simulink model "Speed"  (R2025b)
settings: Solver=FixedStepAuto  StartTime=0.0  StopTime=10.0  FixedStep=1e-4  RelTol=1e-3
undefined symbols (not defined in the file): case, constant, DiscIntNeverNeededParam, flux, lambda_pm, linkage, Permanent, Pn, sigbuilder_block, spd_ki, spd_kp
libraries: slpidlib x3, mcbplantlib x1, autolibpmsmexterior x1

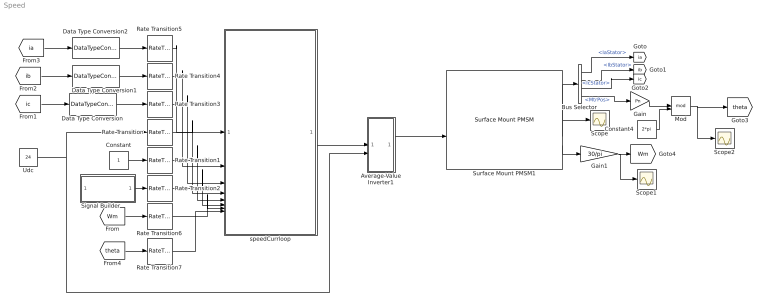
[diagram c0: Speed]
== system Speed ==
  Average-Value Inverter1 : Subsystem
  Bus Selector : BusSelector  OutputSignals=IaStator,IbStator,IcStator,MtrPos
  Constant : Constant
  Constant4 : Constant  Value=2*pi  OutDataTypeStr=Inherit: Inherit via back propagation
  Data Type Conversion : DataTypeConversion  OutDataTypeStr=single
  Data Type Conversion1 : DataTypeConversion  OutDataTypeStr=single
  Data Type Conversion2 : DataTypeConversion  OutDataTypeStr=single
  Gain : Gain  Gain=Pn
  Gain1 : Gain  Gain=30/pi  OutDataTypeStr=single
  Mod : Math  Operator=mod
  Rate Transition{,1..7} (8 alike) : RateTransition
  Scope : Scope
  Scope1 : Scope
  Scope2 : Scope
  Signal Builder : Subsystem  Tag=STV Subsys  LoadFcn=sigbuilder_block('load');  StartFcn=sigbuilder_block('start');  StopFcn=sigbuilder_block('stop');  ClipboardFcn=sigbuilder_block('clipboard');  mask(Sigbuilder block){tuvar=[0:10]}
      mask init:
      | if ~strcmp(get_param(bdroot(gcb),'SimulationStatus'),'stopped'),tuvar = sigbuilder_block('maskInit'); end
  Surface Mount PMSM1 : autolibpmsmexterior/Surface Mount PMSM  port_config=Torque  sim_type=Continuous  Ts=0.001  P=Pn  Rs=Rs  Ldq_=L  KConstText=Permanent flux linkage constant (lambda_pm):  lambda_pm=flux  Ke=159.9771  Kt=1.323  mechanical=[75e-6,8e-5,0]  idq0=[0 0]  theta_init=0  omega_init=0  KConst=0.2205  lambda_pm_calc=0.2205  RefBlkName='autolibpmsmexterior/Surface Mount PMSM'  aMode=5  Ldq="[0.0017      0.0017]"
  Udc : Constant  Value=24
  speedCurrloop : Subsystem
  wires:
  [ia] -> Data Type Conversion2/1
  [ib] -> Data Type Conversion1/1
  [ic] -> Data Type Conversion/1
  Data Type Conversion2/1 -> Rate Transition5/1
  Data Type Conversion1/1 -> Rate Transition4/1
  Data Type Conversion/1 -> Rate Transition3/1
  Udc/1 -> Average-Value Inverter1/2(udc), Rate Transition/1
  Average-Value Inverter1/1(vabc) -> Surface Mount PMSM1/2
  Surface Mount PMSM1/2 -> Scope/1
  Surface Mount PMSM1/1 -> Bus Selector/1
  Bus Selector/1 -> [ia]  "<IaStator>"
  Bus Selector/2 -> [ib]  "<IbStator>"
  Bus Selector/3 -> [ic]  "<IcStator>"
  Bus Selector/4 -> Gain/1  "<MtrPos>"
  Gain/1 -> Mod/1
  Constant4/1 -> Mod/2
  Mod/1 -> Scope2/1, [theta]
  Rate Transition5/1 -> speedCurrloop/1(ia)
  Rate Transition4/1 -> speedCurrloop/2(ib)
  Rate Transition3/1 -> speedCurrloop/3(ic)
  Rate Transition/1 -> speedCurrloop/4(v_bus)
  Constant/1 -> Rate Transition1/1
  speedCurrloop/1(IABC1) -> Average-Value Inverter1/1(Dutyln)
  Rate Transition1/1 -> speedCurrloop/5(Motor_OnOff)
  Rate Transition2/1 -> speedCurrloop/6(SpeedRef)
  Rate Transition6/1 -> speedCurrloop/7(SpeedFd)
  Signal Builder/1(Signal 1) -> Rate Transition2/1
  Surface Mount PMSM1/3 -> Gain1/1
  Gain1/1 -> Scope1/1, [Wm]
  [Wm] -> Rate Transition6/1
  Rate Transition7/1 -> speedCurrloop/8(theta)
  [theta] -> Rate Transition7/1

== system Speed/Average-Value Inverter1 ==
  Dutyln : Inport
  udc : Inport  Port=2
  Average-Value Inverter : mcbplantlib/Average-Value Inverter
  Duty : Subsystem
  vabc : Outport
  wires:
  Dutyln/1 -> Duty/1(Dutyln)
  Duty/1(DutyOut) -> Average-Value Inverter/1
  udc/1 -> Average-Value Inverter/2
  Average-Value Inverter/1 -> vabc/1

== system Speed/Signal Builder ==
  Demux : Demux  Tag=STV Demux  Outputs=1
  FromWs : FromWorkspace  Tag=STV FromWs  VariableName=tuvar
  Signal 1 : Outport  Tag=STV Outport
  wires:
  FromWs/1 -> Demux/1
  Demux/1 -> Signal 1/1

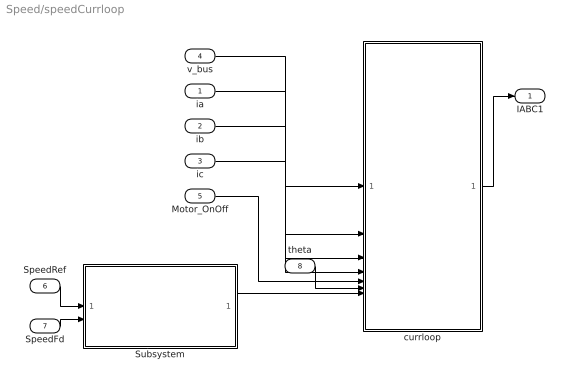
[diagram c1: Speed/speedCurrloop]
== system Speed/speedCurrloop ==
  ia : Inport
  ib : Inport  Port=2
  ic : Inport  Port=3
  v_bus : Inport  Port=4
  Motor_OnOff : Inport  Port=5
  SpeedRef : Inport  Port=6
  SpeedFd : Inport  Port=7
  theta : Inport  Port=8
  Subsystem : Subsystem
  currloop : Subsystem
  IABC1 : Outport
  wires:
  ic/1 -> currloop/4(ic)
  Subsystem/1(iq_ref) -> currloop/7(iq_ref)
  v_bus/1 -> currloop/1(v_bus)
  SpeedRef/1 -> Subsystem/1(SpeedRef)
  ib/1 -> currloop/3(ib)
  currloop/1(IABC1) -> IABC1/1
  Motor_OnOff/1 -> currloop/5(Motor_OnOff)
  ia/1 -> currloop/2(ia)
  SpeedFd/1 -> Subsystem/2(SpeedFd)
  theta/1 -> currloop/6(theta)

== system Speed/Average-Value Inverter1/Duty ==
  Dutyln : Inport
  Subsystem : Subsystem
  DutyOut : Outport
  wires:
  Dutyln/1 -> Subsystem/1(Dutyln)
  Subsystem/1(DutyOut) -> DutyOut/1

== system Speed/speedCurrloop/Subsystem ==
  SpeedRef : Inport
  SpeedFd : Inport  Port=2
  PID Controller : slpidlib/PID Controller  Controller=PI  Form=Parallel  TimeDomain=Discrete-time  UseExternalTs=off  SampleTime=-1  IntegratorMethod=Forward Euler  FilterMethod=Forward Euler  ControllerParametersSource=internal  P=spd_kp  I=spd_ki  UseKiTs=off  D=0  UseExternalDerivativeSource=off  N=100  UseFilter=on  TunerSelectOption=Transfer Function Based (PID Tuner App)  InitialConditionSource=internal  InitialConditionForIntegrator=0  InitialConditionForFilter=0  DifferentiatorICPrevScaledInput=0  ExternalReset=none  TrackingMode=off  Kt=1  LimitOutput=on  SatLimitsSource=internal  UpperSaturationLimit=3  LowerSaturationLimit=-3  LinearizeAsGain=on  AntiWindupMode=clamping  Kb=1  LimitIntegrator=off  UpperIntegratorSaturationLimit=inf  LowerIntegratorSaturationLimit=-inf  POutMin=[]  POutMax=[]  IOutMin=[]  IOutMax=[]  DOutMin=[]  DOutMax=[]  NOutMin=[]  NOutMax=[]  SumOutMin=[]  SumOutMax=[]  SaturationOutMin=[]  SaturationOutMax=[]  PParamMin=[]  PParamMax=[]  IParamMin=[]  IParamMax=[]  DParamMin=[]  DParamMax=[]  NParamMin=[]  NParamMax=[]  KbParamMin=[]  KbParamMax=[]  KtParamMin=[]  KtParamMax=[]  KbOutMin=[]  KbOutMax=[]  KtOutMin=[]  KtOutMax=[]  IntegratorOutMin=[]  IntegratorOutMax=[]  FilterOutMin=[]  FilterOutMax=[]  SumI1OutMin=[]  SumI1OutMax=[]  SumI2OutMin=[]  SumI2OutMax=[]  SumI3OutMin=[]  SumI3OutMax=[]  SumI4OutMin=[]  SumI4OutMax=[]  SumDOutMin=[]  SumDOutMax=[]  DifferentiatorOutMin=[]  DifferentiatorOutMax=[]  FilterDiffOutCoefMin=[]  FilterDiffOutCoefMax=[]  ReciprocalOutMin=[]  ReciprocalOutMax=[]  SumDenOutMin=[]  SumDenOutMax=[]  SumNumOutMin=[]  SumNumOutMax=[]  DivideOutMin=[]  DivideOutMax=[]  UdiffTsProdOutMin=[]  UdiffTsProdOutMax=[]  NTsProdOutMin=[]  NTsProdOutMax=[]  UintegralTsProdOutMin=[]  UintegralTsProdOutMax=[]  UngainTsProdOutMin=[]  UngainTsProdOutMax=[]  ClampingZeroOutDataTypeStr=Inherit: Inherit via back propagation  ClampingZeroOutMin=[]  ClampingZeroOutMax=[]  FilterDenConstantOutDataTypeStr=Inherit: Inherit via back propagation  FilterDenConstantOutMin=[]  FilterDenConstantOutMax=[]  PCopyOutDataTypeStr=Inherit: Inherit via back propagation  PCopyOutMin=[]  PCopyOutMax=[]  NCopyOutDataTypeStr=Inherit: Inherit via back propagation  NCopyOutMin=[]  NCopyOutMax=[]  IntegratorContinuousStateAttributes=''  IntegratorStateMustResolveToSignalObject=off  IntegratorRTWStateStorageClass=Auto  FilterContinuousStateAttributes=''  FilterStateMustResolveToSignalObject=off  FilterRTWStateStorageClass=Auto  ParallelPVariant=InternalParameters  IdealPVariant=Disabled  IVariant=InternalParameters  DVariant=Disabled  IntegratorVariant=Discrete  SatVariant=Enabled  AWVariant=DiscClampingParallel  PCopyVariant=Disabled  TRVariant=Disabled  FdbkBlocksVariant=Forward  IdealPFdbkVariant=Disabled  SatFdbkVariant=Disabled  DerivativeFilterVariant=Disabled  NVariant=Disabled  NCopyVariant=Disabled_SignalSpec  FilterICVariant=Disabled  IntegratorICVariant=InternalICs  ExternalResetVariant=Disabled  TRSumVariant=Passthrough  SumFdbkVariant=Disabled  SumVariant=Sum_PI  TsampFilterVariant=InternalTs  TsampNgainVariant=Passthrough  TsampIntegralVariant=Disabled_SignalSpec  ExternalSaturationOutDataTypeStr=Inherit: Same as second input  DerivativeSourceVariant=Disabled  PreIntVariant=InternalPreInt
  Sum : Sum  Inputs=|+-
  iq_ref : Outport
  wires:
  Sum/1 -> PID Controller/1
  SpeedRef/1 -> Sum/1
  SpeedFd/1 -> Sum/2
  PID Controller/1 -> iq_ref/1

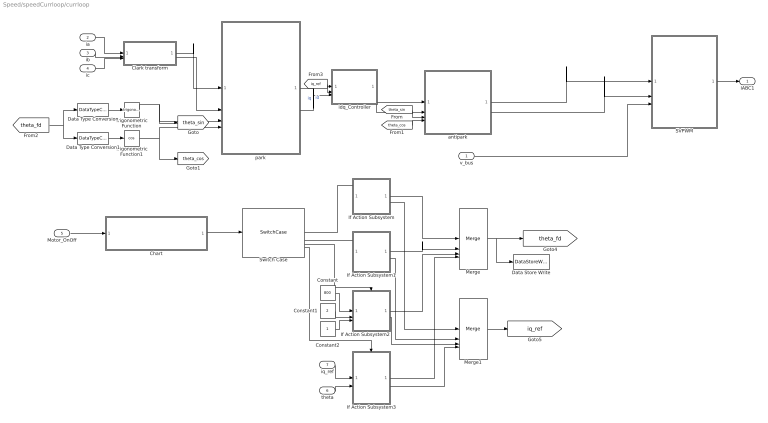
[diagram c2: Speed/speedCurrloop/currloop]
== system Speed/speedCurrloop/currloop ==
  v_bus : Inport
  ia : Inport  Port=2
  ib : Inport  Port=3
  ic : Inport  Port=4
  Motor_OnOff : Inport  Port=5
  theta : Inport  Port=6
  iq_ref : Inport  Port=7
  Chart : Stateflow chart  TreatAsAtomicUnit=on
  Clark transform : Subsystem
  Constant : Constant  Value=800
  Constant1 : Constant  Value=2
  Constant2 : Constant
  Data Store Write : DataStoreWrite  DataStoreName=ThetaOpen  IndexOptions=Index vector (dialog)  Indices=1  OutputSizes=1
  Data Type Conversion : DataTypeConversion  OutDataTypeStr=single
  Data Type Conversion1 : DataTypeConversion  OutDataTypeStr=single
  If Action Subsystem : Subsystem  TreatAsAtomicUnit=on
  If Action Subsystem1 : Subsystem  TreatAsAtomicUnit=on
  If Action Subsystem2 : Subsystem  TreatAsAtomicUnit=on
  If Action Subsystem3 : Subsystem  TreatAsAtomicUnit=on
  Merge : Merge  Inputs=4
  Merge1 : Merge  Inputs=4
  SVPWM : Subsystem
  Switch Case : SwitchCase  CaseConditions={1,2,3,4}  ShowDefaultCase=off
  Trigonometric Function : Trigonometry
  Trigonometric Function1 : Trigonometry  Operator=cos
  antipark : Subsystem
  idq_Controller : Subsystem
  park : Subsystem
  IABC1 : Outport
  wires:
  Clark transform/2(ibeta) -> park/2(ibeta)
  Trigonometric Function1/1 -> [theta_cos], park/4(theta_cos)
  park/1(id) -> idq_Controller/1(id_fdbk)  "id"
  Trigonometric Function/1 -> [theta_sin], park/3(theta_sin)
  idq_Controller/2(uq_ref) -> antipark/2(uq)
  [theta_cos] -> antipark/4(theta_cos)
  Clark transform/1(ialpha) -> park/1(ialpha)
  [theta_fd] -> Data Type Conversion1/1, Data Type Conversion/1
  Data Type Conversion/1 -> Trigonometric Function/1
  park/2(iq) -> idq_Controller/3(iq_fdbk)  "iq"
  [theta_sin] -> antipark/3(theta_sin)
  SVPWM/1(IABC) -> IABC1/1
  antipark/2(ubeta) -> SVPWM/2(Vbeta)
  ic/1 -> Clark transform/3(ic)
  antipark/1(ualpha) -> SVPWM/1(Valpha)
  Data Type Conversion1/1 -> Trigonometric Function1/1
  idq_Controller/1(ud_ref) -> antipark/1(ud)
  v_bus/1 -> SVPWM/3(v_bus)
  ib/1 -> Clark transform/2(ib)
  [iq_ref] -> idq_Controller/2(iq_ref)
  ia/1 -> Clark transform/1(ia)
  If Action Subsystem2/1(theta_fd) -> Merge/3
  Merge/1 -> Data Store Write/1, [theta_fd]
  If Action Subsystem/2(iq_ref) -> Merge1/1
  If Action Subsystem1/1(theta__fd) -> Merge/2
  Switch Case/4 -> If Action Subsystem3/Action
  Constant2/1 -> If Action Subsystem2/3(iq_ref)
  Switch Case/1 -> If Action Subsystem/Action
  If Action Subsystem3/1(theta_fd) -> Merge/4
  If Action Subsystem2/2(iq_fd) -> Merge1/3
  Chart/1(Motor_state) -> Switch Case/1
  Switch Case/3 -> If Action Subsystem2/Action
  Constant/1 -> If Action Subsystem2/1(OPSpd)
  If Action Subsystem1/2(iq_ref) -> Merge1/2
  Merge1/1 -> [iq_ref]
  If Action Subsystem/1(theta_fd) -> Merge/1
  If Action Subsystem3/2(iq_fd) -> Merge1/4
  Switch Case/2 -> If Action Subsystem1/Action
  Constant1/1 -> If Action Subsystem2/2(OPTime)
  Motor_OnOff/1 -> Chart/1(Motor_OnOff)
  iq_ref/1 -> If Action Subsystem3/1(iq_ref)
  theta/1 -> If Action Subsystem3/2(theta)

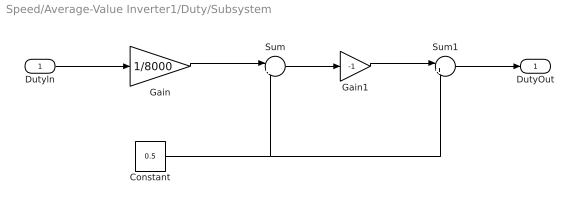
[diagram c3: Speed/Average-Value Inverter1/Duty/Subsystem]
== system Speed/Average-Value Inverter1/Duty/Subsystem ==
  Dutyln : Inport
  Constant : Constant  Value=0.5
  Gain : Gain  Gain=1/8000
  Gain1 : Gain  Gain=-1
  Sum : Sum  Inputs=|+-
  Sum1 : Sum  Inputs=|++
  DutyOut : Outport
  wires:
  Dutyln/1 -> Gain/1
  Constant/1 -> Sum/2, Sum1/2
  Sum1/1 -> DutyOut/1
  Gain/1 -> Sum/1
  Gain1/1 -> Sum1/1
  Sum/1 -> Gain1/1

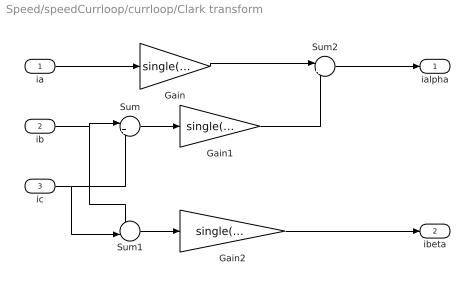
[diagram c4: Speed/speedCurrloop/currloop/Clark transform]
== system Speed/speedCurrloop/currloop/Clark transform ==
  ia : Inport
  ib : Inport  Port=2
  ic : Inport  Port=3
  Gain : Gain  Gain=single(2/3)
  Gain1 : Gain  Gain=single(1/3)
  Gain2 : Gain  Gain=single(sqrt(3)/3)
  Sum : Sum  Inputs=|++
  Sum1 : Sum  Inputs=+-|
  Sum2 : Sum  Inputs=|+-
  ialpha : Outport
  ibeta : Outport  Port=2
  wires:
  ia/1 -> Gain/1
  ib/1 -> Sum1/1, Sum/1
  ic/1 -> Sum1/2, Sum/2
  Sum/1 -> Gain1/1
  Sum1/1 -> Gain2/1
  Gain/1 -> Sum2/1
  Gain1/1 -> Sum2/2
  Gain2/1 -> ibeta/1
  Sum2/1 -> ialpha/1

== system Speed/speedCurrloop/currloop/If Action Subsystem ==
  Action Port : ActionPort  ActionPortLabel=case [ 1 ]:
  Constant : Constant  Value=0
  Constant1 : Constant  Value=0
  theta_fd : Outport
  iq_ref : Outport  Port=2
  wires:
  Constant/1 -> theta_fd/1
  Constant1/1 -> iq_ref/1

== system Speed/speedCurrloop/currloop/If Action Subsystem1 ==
  Action Port : ActionPort  ActionPortLabel=case [ 2 ]:
  Constant : Constant  Value=0
  Constant1 : Constant
  theta__fd : Outport
  iq_ref : Outport  Port=2
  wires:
  Constant/1 -> theta__fd/1
  Constant1/1 -> iq_ref/1

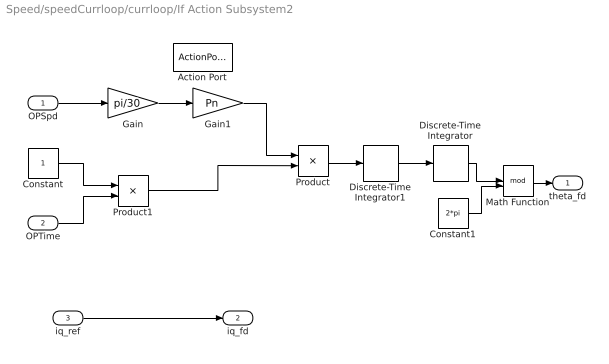
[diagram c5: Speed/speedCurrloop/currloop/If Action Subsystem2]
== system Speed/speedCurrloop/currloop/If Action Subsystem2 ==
  OPSpd : Inport
  OPTime : Inport  Port=2
  iq_ref : Inport  Port=3
  Action Port : ActionPort  ActionPortLabel=case [ 3 ]:
  Constant : Constant
  Constant1 : Constant  Value=2*pi
  Discrete-Time Integrator : DiscreteIntegrator  SampleTime=-1  ICPrevOutput=DiscIntNeverNeededParam  ICPrevScaledInput=DiscIntNeverNeededParam
  Discrete-Time Integrator1 : DiscreteIntegrator  SampleTime=-1  ICPrevOutput=DiscIntNeverNeededParam  ICPrevScaledInput=DiscIntNeverNeededParam
  Gain : Gain  Gain=pi/30  OutDataTypeStr=single
  Gain1 : Gain  Gain=Pn
  Math Function : Math  Operator=mod
  Product : Product
  Product1 : Product  Inputs=*/
  theta_fd : Outport
  iq_fd : Outport  Port=2
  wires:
  OPTime/1 -> Product1/2
  Constant/1 -> Product1/1
  Product/1 -> Discrete-Time Integrator1/1
  Gain/1 -> Gain1/1
  Gain1/1 -> Product/1
  Constant1/1 -> Math Function/2
  OPSpd/1 -> Gain/1
  Discrete-Time Integrator/1 -> Math Function/1
  Discrete-Time Integrator1/1 -> Discrete-Time Integrator/1
  Math Function/1 -> theta_fd/1
  Product1/1 -> Product/2
  iq_ref/1 -> iq_fd/1

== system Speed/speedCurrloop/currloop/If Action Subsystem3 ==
  iq_ref : Inport  SampleTime=1e-4
  theta : Inport  Port=2  SampleTime=1e-4
  Action Port : ActionPort  ActionPortLabel=case [ 4 ]:
  theta_fd : Outport  SampleTime=1e-4
  iq_fd : Outport  Port=2  SampleTime=1e-4
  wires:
  theta/1 -> theta_fd/1
  iq_ref/1 -> iq_fd/1

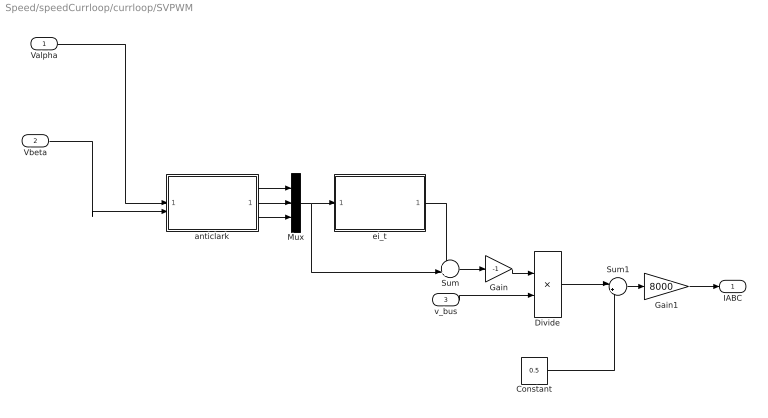
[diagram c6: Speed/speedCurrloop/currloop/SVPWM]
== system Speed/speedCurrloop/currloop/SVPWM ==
  Valpha : Inport
  Vbeta : Inport  Port=2
  v_bus : Inport  Port=3  OutMin=10
  Constant : Constant  Value=0.5
  Divide : Product  Inputs=*/
  Gain : Gain  Gain=-1
  Gain1 : Gain  Gain=8000
  Mux : Mux  Inputs=3
  Sum : Sum  Inputs=++|
  Sum1 : Sum  Inputs=|++
  anticlark : Subsystem
  ei_t : Subsystem
  IABC : Outport
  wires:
  ei_t/1(ei_t1) -> Sum/1
  Gain1/1 -> IABC/1
  anticlark/2(Vb) -> Mux/2
  Vbeta/1 -> anticlark/2(Vbeta)
  Constant/1 -> Sum1/2
  anticlark/3(Vc) -> Mux/3
  Divide/1 -> Sum1/1
  Sum/1 -> Gain/1
  Gain/1 -> Divide/1
  Sum1/1 -> Gain1/1
  anticlark/1(Va) -> Mux/1
  v_bus/1 -> Divide/2
  Mux/1 -> Sum/2, ei_t/1(Vabc)
  Valpha/1 -> anticlark/1(Valpha)

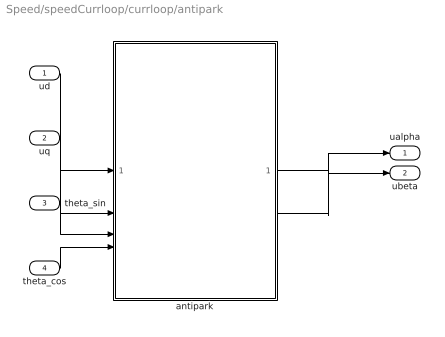
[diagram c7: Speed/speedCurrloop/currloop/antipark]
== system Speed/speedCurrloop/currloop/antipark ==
  ud : Inport
  uq : Inport  Port=2
  theta_sin : Inport  Port=3
  theta_cos : Inport  Port=4
  antipark : Subsystem
  ualpha : Outport
  ubeta : Outport  Port=2
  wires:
  theta_cos/1 -> antipark/4(theta_cos)
  theta_sin/1 -> antipark/3(theta_sin)
  antipark/2(ubeta) -> ubeta/1
  antipark/1(ualpha) -> ualpha/1
  ud/1 -> antipark/1(ud)
  uq/1 -> antipark/2(uq)

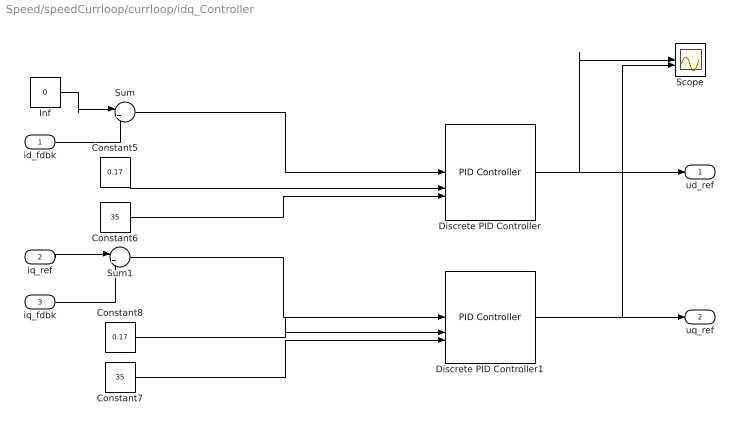
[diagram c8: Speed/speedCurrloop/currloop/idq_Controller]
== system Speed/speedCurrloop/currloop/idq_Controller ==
  id_fdbk : Inport
  iq_ref : Inport  Port=2
  iq_fdbk : Inport  Port=3
  Constant5 : Constant  Value=0.17  OutDataTypeStr=single
  Constant6 : Constant  Value=35  OutDataTypeStr=single
  Constant7 : Constant  Value=35  OutDataTypeStr=single
  Constant8 : Constant  Value=0.17  OutDataTypeStr=single
  Discrete PID Controller : slpidlib/PID Controller  Controller=PI  Form=Parallel  TimeDomain=Discrete-time  UseExternalTs=off  SampleTime=-1  IntegratorMethod=Forward Euler  FilterMethod=Forward Euler  ControllerParametersSource=external  P=1  I=1  UseKiTs=off  D=0  UseExternalDerivativeSource=off  N=100  UseFilter=off  TunerSelectOption=Transfer Function Based (PID Tuner App)  InitialConditionSource=internal  InitialConditionForIntegrator=0  InitialConditionForFilter=0  DifferentiatorICPrevScaledInput=0  ExternalReset=none  TrackingMode=off  Kt=1  LimitOutput=on  SatLimitsSource=internal  UpperSaturationLimit=24*0.9/sqrt(3)  LowerSaturationLimit=-24*0.9/sqrt(3)  LinearizeAsGain=on  AntiWindupMode=clamping  Kb=1  LimitIntegrator=off  UpperIntegratorSaturationLimit=inf  LowerIntegratorSaturationLimit=-inf  POutMin=[]  POutMax=[]  IOutMin=[]  IOutMax=[]  DOutMin=[]  DOutMax=[]  NOutMin=[]  NOutMax=[]  SumOutMin=[]  SumOutMax=[]  SaturationOutMin=[]  SaturationOutMax=[]  PParamMin=[]  PParamMax=[]  IParamMin=[]  IParamMax=[]  DParamMin=[]  DParamMax=[]  NParamMin=[]  NParamMax=[]  KbParamMin=[]  KbParamMax=[]  KtParamMin=[]  KtParamMax=[]  KbOutMin=[]  KbOutMax=[]  KtOutMin=[]  KtOutMax=[]  IntegratorOutMin=[]  IntegratorOutMax=[]  FilterOutMin=[]  FilterOutMax=[]  SumI1OutMin=[]  SumI1OutMax=[]  SumI2OutMin=[]  SumI2OutMax=[]  SumI3OutMin=[]  SumI3OutMax=[]  SumI4OutMin=[]  SumI4OutMax=[]  SumDOutMin=[]  SumDOutMax=[]  DifferentiatorOutMin=[]  DifferentiatorOutMax=[]  FilterDiffOutCoefMin=[]  FilterDiffOutCoefMax=[]  ReciprocalOutMin=[]  ReciprocalOutMax=[]  SumDenOutMin=[]  SumDenOutMax=[]  SumNumOutMin=[]  SumNumOutMax=[]  DivideOutMin=[]  DivideOutMax=[]  UdiffTsProdOutMin=[]  UdiffTsProdOutMax=[]  NTsProdOutMin=[]  NTsProdOutMax=[]  UintegralTsProdOutMin=[]  UintegralTsProdOutMax=[]  UngainTsProdOutMin=[]  UngainTsProdOutMax=[]  ClampingZeroOutDataTypeStr=Inherit: Inherit via back propagation  ClampingZeroOutMin=[]  ClampingZeroOutMax=[]  FilterDenConstantOutDataTypeStr=Inherit: Inherit via back propagation  FilterDenConstantOutMin=[]  FilterDenConstantOutMax=[]  PCopyOutDataTypeStr=Inherit: Inherit via back propagation  PCopyOutMin=[]  PCopyOutMax=[]  NCopyOutDataTypeStr=Inherit: Inherit via back propagation  NCopyOutMin=[]  NCopyOutMax=[]  IntegratorContinuousStateAttributes=''  IntegratorStateMustResolveToSignalObject=off  IntegratorRTWStateStorageClass=Auto  FilterContinuousStateAttributes=''  FilterStateMustResolveToSignalObject=off  FilterRTWStateStorageClass=Auto  ParallelPVariant=ExternalParameters  IdealPVariant=Disabled  IVariant=ExternalParameters  DVariant=Disabled  IntegratorVariant=Discrete  SatVariant=Enabled  AWVariant=DiscClampingParallel  PCopyVariant=Disabled  TRVariant=Disabled  FdbkBlocksVariant=Forward  IdealPFdbkVariant=Disabled  SatFdbkVariant=Disabled  DerivativeFilterVariant=Disabled  NVariant=Disabled  NCopyVariant=Disabled_SignalSpec  FilterICVariant=Disabled  IntegratorICVariant=InternalICs  ExternalResetVariant=Disabled  TRSumVariant=Passthrough  SumFdbkVariant=Disabled  SumVariant=Sum_PI  TsampFilterVariant=InternalTs  TsampNgainVariant=Passthrough  TsampIntegralVariant=Disabled_SignalSpec  ExternalSaturationOutDataTypeStr=Inherit: Same as second input  DerivativeSourceVariant=Disabled  PreIntVariant=InternalPreInt
  Discrete PID Controller1 : slpidlib/PID Controller  Controller=PI  Form=Parallel  TimeDomain=Discrete-time  UseExternalTs=off  SampleTime=-1  IntegratorMethod=Forward Euler  FilterMethod=Forward Euler  ControllerParametersSource=external  P=1  I=1  UseKiTs=off  D=0  UseExternalDerivativeSource=off  N=100  UseFilter=off  TunerSelectOption=Transfer Function Based (PID Tuner App)  InitialConditionSource=internal  InitialConditionForIntegrator=0  InitialConditionForFilter=0  DifferentiatorICPrevScaledInput=0  ExternalReset=none  TrackingMode=off  Kt=1  LimitOutput=on  SatLimitsSource=internal  UpperSaturationLimit=24*0.9/sqrt(3)  LowerSaturationLimit=-24*0.9/sqrt(3)  LinearizeAsGain=off  AntiWindupMode=none  Kb=1  LimitIntegrator=off  UpperIntegratorSaturationLimit=inf  LowerIntegratorSaturationLimit=-inf  POutMin=[]  POutMax=[]  IOutMin=[]  IOutMax=[]  DOutMin=[]  DOutMax=[]  NOutMin=[]  NOutMax=[]  SumOutMin=[]  SumOutMax=[]  SaturationOutMin=[]  SaturationOutMax=[]  PParamMin=[]  PParamMax=[]  IParamMin=[]  IParamMax=[]  DParamMin=[]  DParamMax=[]  NParamMin=[]  NParamMax=[]  KbParamMin=[]  KbParamMax=[]  KtParamMin=[]  KtParamMax=[]  KbOutMin=[]  KbOutMax=[]  KtOutMin=[]  KtOutMax=[]  IntegratorOutMin=[]  IntegratorOutMax=[]  FilterOutMin=[]  FilterOutMax=[]  SumI1OutMin=[]  SumI1OutMax=[]  SumI2OutMin=[]  SumI2OutMax=[]  SumI3OutMin=[]  SumI3OutMax=[]  SumI4OutMin=[]  SumI4OutMax=[]  SumDOutMin=[]  SumDOutMax=[]  DifferentiatorOutMin=[]  DifferentiatorOutMax=[]  FilterDiffOutCoefMin=[]  FilterDiffOutCoefMax=[]  ReciprocalOutMin=[]  ReciprocalOutMax=[]  SumDenOutMin=[]  SumDenOutMax=[]  SumNumOutMin=[]  SumNumOutMax=[]  DivideOutMin=[]  DivideOutMax=[]  UdiffTsProdOutMin=[]  UdiffTsProdOutMax=[]  NTsProdOutMin=[]  NTsProdOutMax=[]  UintegralTsProdOutMin=[]  UintegralTsProdOutMax=[]  UngainTsProdOutMin=[]  UngainTsProdOutMax=[]  ClampingZeroOutDataTypeStr=Inherit: Inherit via back propagation  ClampingZeroOutMin=[]  ClampingZeroOutMax=[]  FilterDenConstantOutDataTypeStr=Inherit: Inherit via back propagation  FilterDenConstantOutMin=[]  FilterDenConstantOutMax=[]  PCopyOutDataTypeStr=Inherit: Inherit via back propagation  PCopyOutMin=[]  PCopyOutMax=[]  NCopyOutDataTypeStr=Inherit: Inherit via back propagation  NCopyOutMin=[]  NCopyOutMax=[]  IntegratorContinuousStateAttributes=''  IntegratorStateMustResolveToSignalObject=off  IntegratorRTWStateStorageClass=Auto  FilterContinuousStateAttributes=''  FilterStateMustResolveToSignalObject=off  FilterRTWStateStorageClass=Auto  ParallelPVariant=ExternalParameters  IdealPVariant=Disabled  IVariant=ExternalParameters  DVariant=Disabled  IntegratorVariant=Discrete  SatVariant=Enabled  AWVariant=Passthrough  PCopyVariant=Disabled  TRVariant=Disabled  FdbkBlocksVariant=Forward  IdealPFdbkVariant=Disabled  SatFdbkVariant=Disabled  DerivativeFilterVariant=Disabled  NVariant=Disabled  NCopyVariant=Disabled_SignalSpec  FilterICVariant=Disabled  IntegratorICVariant=InternalICs  ExternalResetVariant=Disabled  TRSumVariant=Passthrough  SumFdbkVariant=Disabled  SumVariant=Sum_PI  TsampFilterVariant=InternalTs  TsampNgainVariant=Passthrough  TsampIntegralVariant=Disabled_SignalSpec  ExternalSaturationOutDataTypeStr=Inherit: Same as second input  DerivativeSourceVariant=Disabled  PreIntVariant=InternalPreInt
  Inf : Constant  Value=0
  Scope : Scope  NumInputPorts=2
  Sum : Sum  Inputs=|++
  Sum1 : Sum  Inputs=|++
  ud_ref : Outport
  uq_ref : Outport  Port=2
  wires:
  Sum1/1 -> Discrete PID Controller1/1
  Discrete PID Controller1/1 -> uq_ref/1, Scope/2
  Constant5/1 -> Discrete PID Controller/2
  id_fdbk/1 -> Sum/2
  Constant8/1 -> Discrete PID Controller1/2
  Constant7/1 -> Discrete PID Controller1/3
  Discrete PID Controller/1 -> ud_ref/1, Scope/1
  Constant6/1 -> Discrete PID Controller/3
  iq_fdbk/1 -> Sum1/2
  Inf/1 -> Sum/1
  Sum/1 -> Discrete PID Controller/1
  iq_ref/1 -> Sum1/1

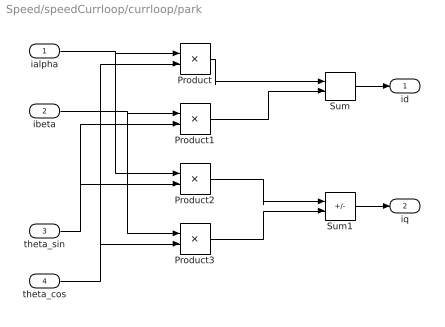
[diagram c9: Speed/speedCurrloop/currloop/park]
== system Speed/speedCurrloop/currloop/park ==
  ialpha : Inport
  ibeta : Inport  Port=2
  theta_sin : Inport  Port=3
  theta_cos : Inport  Port=4
  Product{,1..3} (4 alike) : Product
  Sum : Sum  Inputs=|++
  Sum1 : Sum  Inputs=|-+
  id : Outport
  iq : Outport  Port=2
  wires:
  ialpha/1 -> Product2/1, Product/1
  ibeta/1 -> Product1/1, Product3/1
  theta_sin/1 -> Product1/2, Product2/2
  theta_cos/1 -> Product3/2, Product/2
  Product/1 -> Sum/1
  Product1/1 -> Sum/2
  Product2/1 -> Sum1/1
  Product3/1 -> Sum1/2
  Sum1/1 -> iq/1
  Sum/1 -> id/1

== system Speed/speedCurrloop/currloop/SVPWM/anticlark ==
  Valpha : Inport
  Vbeta : Inport  Port=2
  anticlark : Subsystem
  Va : Outport
  Vb : Outport  Port=2
  Vc : Outport  Port=3
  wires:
  anticlark/3(Vc) -> Vc/1
  Vbeta/1 -> anticlark/2(Vbeta)
  anticlark/1(Va) -> Va/1
  anticlark/2(Vb) -> Vb/1
  Valpha/1 -> anticlark/1(Valpha)

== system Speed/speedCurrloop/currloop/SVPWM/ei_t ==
  Vabc : Inport
  ei_t : Subsystem
  ei_t1 : Outport
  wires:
  Vabc/1 -> ei_t/1(Vabc)
  ei_t/1(ei_t) -> ei_t1/1

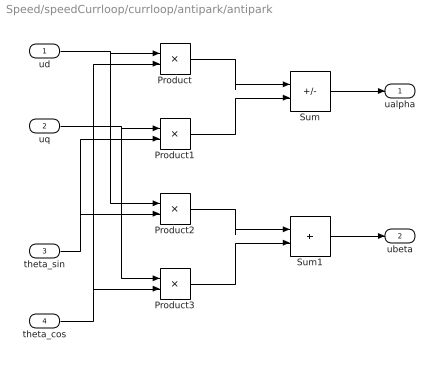
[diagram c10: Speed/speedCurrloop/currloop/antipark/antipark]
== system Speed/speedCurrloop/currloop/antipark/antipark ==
  ud : Inport
  uq : Inport  Port=2
  theta_sin : Inport  Port=3
  theta_cos : Inport  Port=4
  Product{,1..3} (4 alike) : Product
  Sum : Sum  Inputs=|+-
  Sum1 : Sum  Inputs=|++
  ualpha : Outport
  ubeta : Outport  Port=2
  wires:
  theta_cos/1 -> Product3/2, Product/2
  theta_sin/1 -> Product1/2, Product2/2
  uq/1 -> Product3/1, Product1/1
  ud/1 -> Product2/1, Product/1
  Product/1 -> Sum/1
  Product1/1 -> Sum/2
  Product2/1 -> Sum1/1
  Product3/1 -> Sum1/2
  Sum/1 -> ualpha/1
  Sum1/1 -> ubeta/1

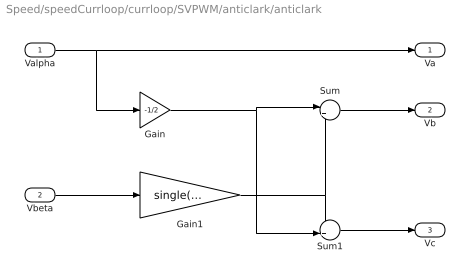
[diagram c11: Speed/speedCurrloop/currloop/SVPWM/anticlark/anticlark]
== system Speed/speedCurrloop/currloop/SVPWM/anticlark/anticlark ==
  Valpha : Inport
  Vbeta : Inport  Port=2
  Gain : Gain  Gain=-1/2
  Gain1 : Gain  Gain=single(sqrt(3)/2)
  Sum : Sum  Inputs=|++
  Sum1 : Sum  Inputs=-+|
  Va : Outport
  Vb : Outport  Port=2
  Vc : Outport  Port=3
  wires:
  Valpha/1 -> Gain/1, Va/1
  Gain/1 -> Sum1/2, Sum/1
  Gain1/1 -> Sum1/1, Sum/2
  Sum/1 -> Vb/1
  Vbeta/1 -> Gain1/1
  Sum1/1 -> Vc/1

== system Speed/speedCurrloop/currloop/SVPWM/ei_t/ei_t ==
  Vabc : Inport
  Demux : Demux  Outputs=3
  Gain : Gain  Gain=-1/2
  MinMax : MinMax  Inputs=3
  MinMax1 : MinMax  Function=max  Inputs=3
  Sum : Sum  Inputs=|++
  ei_t : Outport
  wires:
  Vabc/1 -> Demux/1
  Demux/1 -> MinMax1/1, MinMax/1
  Demux/2 -> MinMax1/2, MinMax/2
  Demux/3 -> MinMax1/3, MinMax/3
  MinMax/1 -> Sum/1
  MinMax1/1 -> Sum/2
  Sum/1 -> Gain/1
  Gain/1 -> ei_t/1

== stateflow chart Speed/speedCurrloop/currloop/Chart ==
  state OpenStage
    en:
    du:
    Motor_state = 3;
  state RunStage
    en:
    du:
    Motor_state = 4;
  state IDLE
    en:
    du:
    Motor_state = 1;
  state AlignStage
    en:
    du:
    Motor_state = 2;
  AlignStage -> OpenStage : [[after(1000, tick)]]
  IDLE -> AlignStage : [Motor_OnOff == 1]
  OpenStage -> RunStage : [[after(30000, tick)]]
  (default) -> IDLE
  OpenStage -> IDLE : [Motor_OnOff == 0]
  RunStage -> IDLE : [Motor_OnOff == 0]
  AlignStage -> IDLE : [Motor_OnOff == 0]
  data: Motor_OnOff input; Motor_state output
